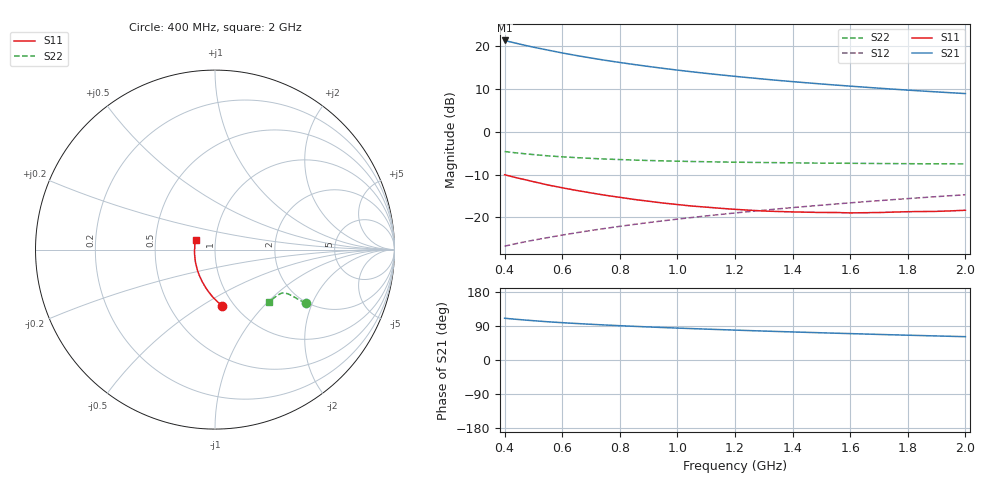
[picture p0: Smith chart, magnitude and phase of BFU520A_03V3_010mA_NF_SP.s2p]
! Filename:  P:\Prog\Test\Noise\ATS_data\Testdata_Net\06 Compressed Noise after Statistics\BFU520A_APG2013_30_A05_03p3V_010mA_NF_CM01_D.sf
! Date/Time: Wed 24/Apr/2013 20:06:16
! BFU520A_APG2013_30_A05_03p3V_1to20mA_NF_CM01_Bias6_R.sf
! Noise Parameter Data File
! BFU520A_APG2013_30_A05_03p3V_1to20mA_NF_CM01
! Date/time: Thu Apr 11 00:04:13 2013
! VAR V_out= 3.300000
! VAR I_out= 10.000000
! VAR V_in= 0.847900
! VAR I_in= 0.113400
! Device data file deembeded for feedlines and parallel
! Original file: \06 Compressed Noise after Statistics\BFU520A_APG2013_30_A05_03p3V_010mA_NF_CM01_R.sf
! Feed-files: PR017V01_150413_Feed1.s2p, PR017V01_150413_Feed2.s2p
! Parallel-file: PR017V01_150413_Par.s2p
# MHz S MA R 50
!  Freq-MHz  S11-mag  S11-arg  S21-mag  S21-arg  S12-mag  S12-arg  S22-mag  S22-arg
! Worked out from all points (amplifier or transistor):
!   37 points, 400 MHz to 2 GHz, reference 50 ohm
!   highest |S21| = 21.2 dB at 400 MHz (marker M1)
!   |S21| within 3 dB of that: start of sweep to 607.8 MHz
!   unconditionally stable (mu >= 1): 1.209 GHz to end of sweep
!   at 500 MHz: K = 0.83, MSG = 22.5 dB, |S12| = -25.3 dB
!   at 1.1 GHz: K = 0.99, MSG = 16.6 dB, |S12| = -19.6 dB
!   at 2 GHz: K = 1.01, MAG = 11.3 dB, |S12| = -14.7 dB
!   lowest NFmin = 0.84 dB at 420 MHz
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400  0.3141 -82.9  11.47 110.3  0.04636 68.1  0.5853 -30.5
420  0.3023 -85.1  11.04 108.8  0.04798 68.2  0.5743 -30.6
440  0.2906 -87.3  10.64 107.4  0.04962 68.3  0.5646 -30.7
460  0.2805 -89.3  10.26 106.1  0.05119 68.4  0.5557 -30.8
480  0.2709 -91.4  9.913 104.9  0.05278 68.5  0.5468 -30.9
500  0.261 -93.4  9.582 103.7  0.05439 68.6  0.5394 -30.9
550  0.239 -98.3  8.864 100.9  0.05832 69.0  0.5212 -30.9
600  0.2216 -102.8  8.209 98.5  0.06239 69.3  0.508 -30.9
650  0.2062 -107.1  7.657 96.3  0.06644 69.6  0.4964 -31.1
700  0.1932 -111.4  7.171 94.2  0.07056 69.9  0.4868 -31.1
750  0.1812 -115.6  6.738 92.3  0.07469 70.2  0.4785 -31.2
800  0.1714 -119.9  6.36 90.5  0.07886 70.4  0.4718 -31.4
850  0.162 -124.2  6.02 88.8  0.08301 70.5  0.4655 -31.6
950  0.1472 -132.3  5.435 85.7  0.09143 70.8  0.4559 -32.1
1050  0.1358 -140.4  4.957 82.8  0.09987 70.9  0.4481 -32.7
1150  0.1278 -149.0  4.559 80.2  0.1085 70.9  0.4421 -33.5
1200  0.1244 -152.7  4.385 78.9  0.1129 70.9  0.4399 -33.9
1350  0.1174 -164.5  3.934 75.2  0.1259 70.6  0.4342 -35.3
1500  0.1143 -176.2  3.575 71.8  0.139 70.2  0.4288 -37.0
1650  0.1136 173.5  3.281 68.6  0.1525 69.7  0.4258 -38.9
1750  0.1155 167.1  3.11 66.4  0.1613 69.3  0.4235 -40.1
2000  0.1213 153.3  2.764 61.5  0.1838 68.1  0.4198 -43.7
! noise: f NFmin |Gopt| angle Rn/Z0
400  0.8652  0.04571  162.7  0.0992
460  0.8579  0.05396  -172.3  0.0904
600  0.9701  0.02989  -128.5  0.1141
800  0.9101  0.08282  -161.9  0.0912
1000  0.9527  0.08301  -160.7  0.0918
1200  0.9819  0.09452  -154.8  0.0957
1400  1.033  0.122  -148.7  0.0902
1600  1.01  0.1621  -146.5  0.0866
1800  0.9944  0.1971  -146.8  0.0806
2000  1.022  0.1976  -137.7  0.0925
